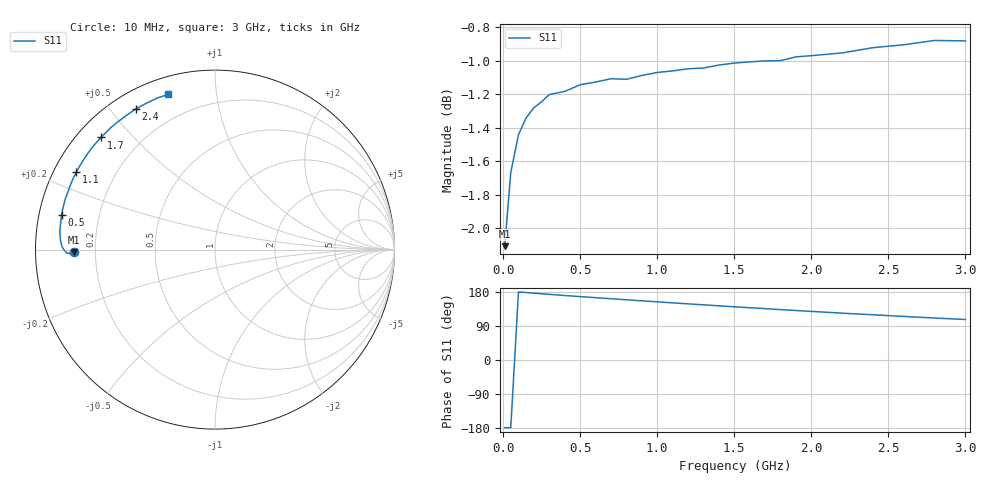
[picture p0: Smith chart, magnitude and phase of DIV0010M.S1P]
! SIEMENS Small Signal Semiconductors
! BAV99
! Silicon Switching Diode in SOT23
! IF = 10 mA
! S-Parameters:  May  1995
# GHz  S  MA  R  50
!  f  S11
! GHz  MAG  ANG
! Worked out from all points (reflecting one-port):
!   30 points, 10 MHz to 3 GHz, reference 50 ohm
!   lowest |S11| = -2.1 dB at 10 MHz (marker M1), VSWR 8.29, Z = 6.03 - j0.43 ohm
!   phase of S11 starts at -179 deg and turns -74 deg over the sweep
!   S11 on the Smith chart (normalised r, x): 10 MHz: 0.12, -0.01; 500 MHz: 0.07, +0.11; 1.1 GHz: 0.07, +0.26; 1.7 GHz: 0.07, +0.41; 2.4 GHz: 0.07, +0.58; 3 GHz: 0.08, +0.74
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0.01  0.7847 -179.0
0.02  0.7942 -178.4
0.05  0.8254 -178.6
0.1  0.8471 179.6
0.15  0.857 178.0
0.2  0.8629 176.4
0.3  0.8708 173.2
0.4  0.8726 170.2
0.5  0.8767 167.3
0.6  0.8782 164.5
0.7  0.8803 161.7
0.8  0.8799 158.9
0.9  0.8822 156.2
1  0.8841 153.5
1.1  0.885 150.8
1.2  0.8863 148.2
1.4  0.8885 143.0
1.5  0.8898 140.4
1.6  0.8905 138.0
1.7  0.8911 135.5
1.8  0.8913 133.0
1.9  0.8936 130.6
2  0.8943 128.3
2.2  0.896 123.6
2.4  0.8992 119.3
2.6  0.901 115.0
2.8  0.9037 110.8
3  0.9034 106.9
